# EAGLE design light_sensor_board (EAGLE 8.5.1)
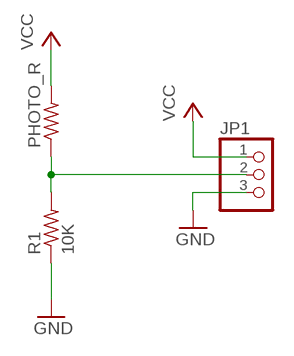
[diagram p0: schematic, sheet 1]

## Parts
JP1  PINHD-1X3  [1X03]
PHOTO_R  R-US_R0805  [R0805]
R1  10K  R-US_R0805  [R0805]

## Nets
GND: JP1.3 R1.1
N$2: JP1.2 PHOTO_R.1 R1.2
VCC: JP1.1 PHOTO_R.2

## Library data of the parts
JP1 = adafruit:PINHD-1X3: PIN HEADER
PHOTO_R R1 = rcl:R-US_: RESISTOR, American symbol; SPICEPREFIX: R

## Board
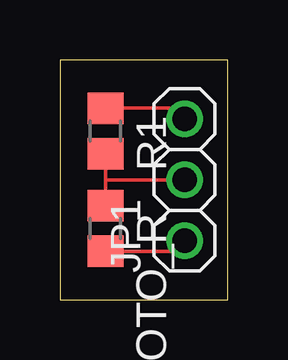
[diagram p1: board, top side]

Size 7 x 10 mm. Coordinates in mm from the lower left corner, seen from the top.
Outline: 0,0 7,0 7,10 0,10 0,0
Copper layers (1*16): Top 0.035mm / dielectric 1.5mm / Bottom 0.035mm
Design rules "default": minimum track width 6mil, minimum drill 0.35mm, track to track 6mil, track to pad 6mil, pad to pad 6mil, via to via 6mil, smd to smd 6mil, copper to edge 40mil, drill to drill 6mil, minimum pad ring 10mil, minimum via ring 8mil, stop-mask expansion 4mil, vias tented up to drill 0mil, thermal gap 10mil

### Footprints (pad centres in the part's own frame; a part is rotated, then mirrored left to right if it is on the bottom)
1X03 = drill 1.016: 1 -2.54,0; 2 0,0; 3 2.54,0
R0805 = smd 1.3 x 1.5: 1 -0.95,0; 2 0.95,0

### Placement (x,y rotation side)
JP1  5.21,5 90 top
PHOTO_R  1.91,2.97 270 top
R1  1.91,7.03 270 top

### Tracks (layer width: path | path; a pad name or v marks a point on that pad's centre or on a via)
GND
  Top 0.152: 2.22,7.67 R1.1 4.76,7.98 JP1.3
N$2
  Top 0.152: R1.2 1.91,5 | 1.91,5 PHOTO_R.1 | JP1.2 1.91,5
VCC
  Top 0.152: PHOTO_R.2 4.76,2.02 JP1.1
